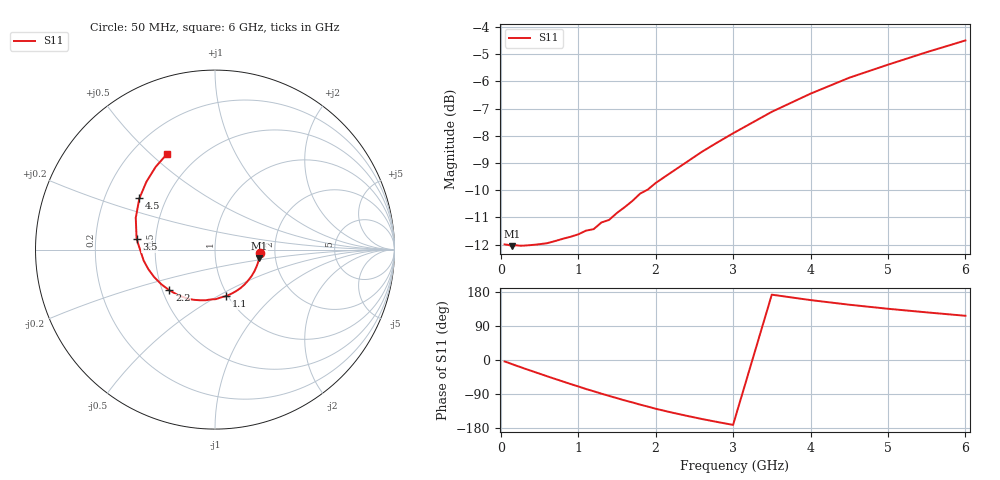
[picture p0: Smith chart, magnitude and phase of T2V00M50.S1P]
! SIEMENS Discrete & RF Semiconductors
! BAS70-04W
! Si Schottky Diode in SOT323
! IF = 0.5 mA
! S-Parameters:  November  1997
# GHz  S  MA  R  50
!  f  S11
! GHz  MAG  ANG
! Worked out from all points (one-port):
!   34 points, 50 MHz to 6 GHz, reference 50 ohm
!   lowest |S11| = -12.1 dB at 150 MHz (marker M1), VSWR 1.66, Z = 81.9 - j8.46 ohm
!   |S11| at or under -10 dB: start of sweep to 1.884 GHz
!   S11 on the Smith chart (normalised r, x): 50 MHz: 1.67, -0.06; 1.1 GHz: 0.98, -0.55; 2.2 GHz: 0.54, -0.28; 3.5 GHz: 0.39, +0.06; 4.5 GHz: 0.35, +0.27; 6 GHz: 0.34, +0.56
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0.05  0.2514 -3.9
0.15  0.2495 -11.2
0.3  0.2501 -22.1
0.5  0.2516 -36.0
0.7  0.2549 -49.8
0.8  0.2574 -56.5
0.9  0.2596 -63.3
1.1  0.2664 -76.5
1.2  0.2682 -82.5
1.3  0.2758 -88.8
1.4  0.2789 -94.8
1.5  0.2871 -100.6
1.6  0.2943 -106.6
1.7  0.3021 -111.9
1.8  0.3117 -117.8
1.9  0.3171 -123.0
2  0.326 -128.6
2.2  0.3408 -138.2
2.4  0.3561 -147.2
2.6  0.3722 -155.8
2.8  0.3872 -163.7
3  0.4023 -171.3
3.5  0.4406 172.4
4  0.4758 158.1
4.5  0.509 145.9
5  0.5379 135.2
5.5  0.5671 125.7
6  0.596 116.7
